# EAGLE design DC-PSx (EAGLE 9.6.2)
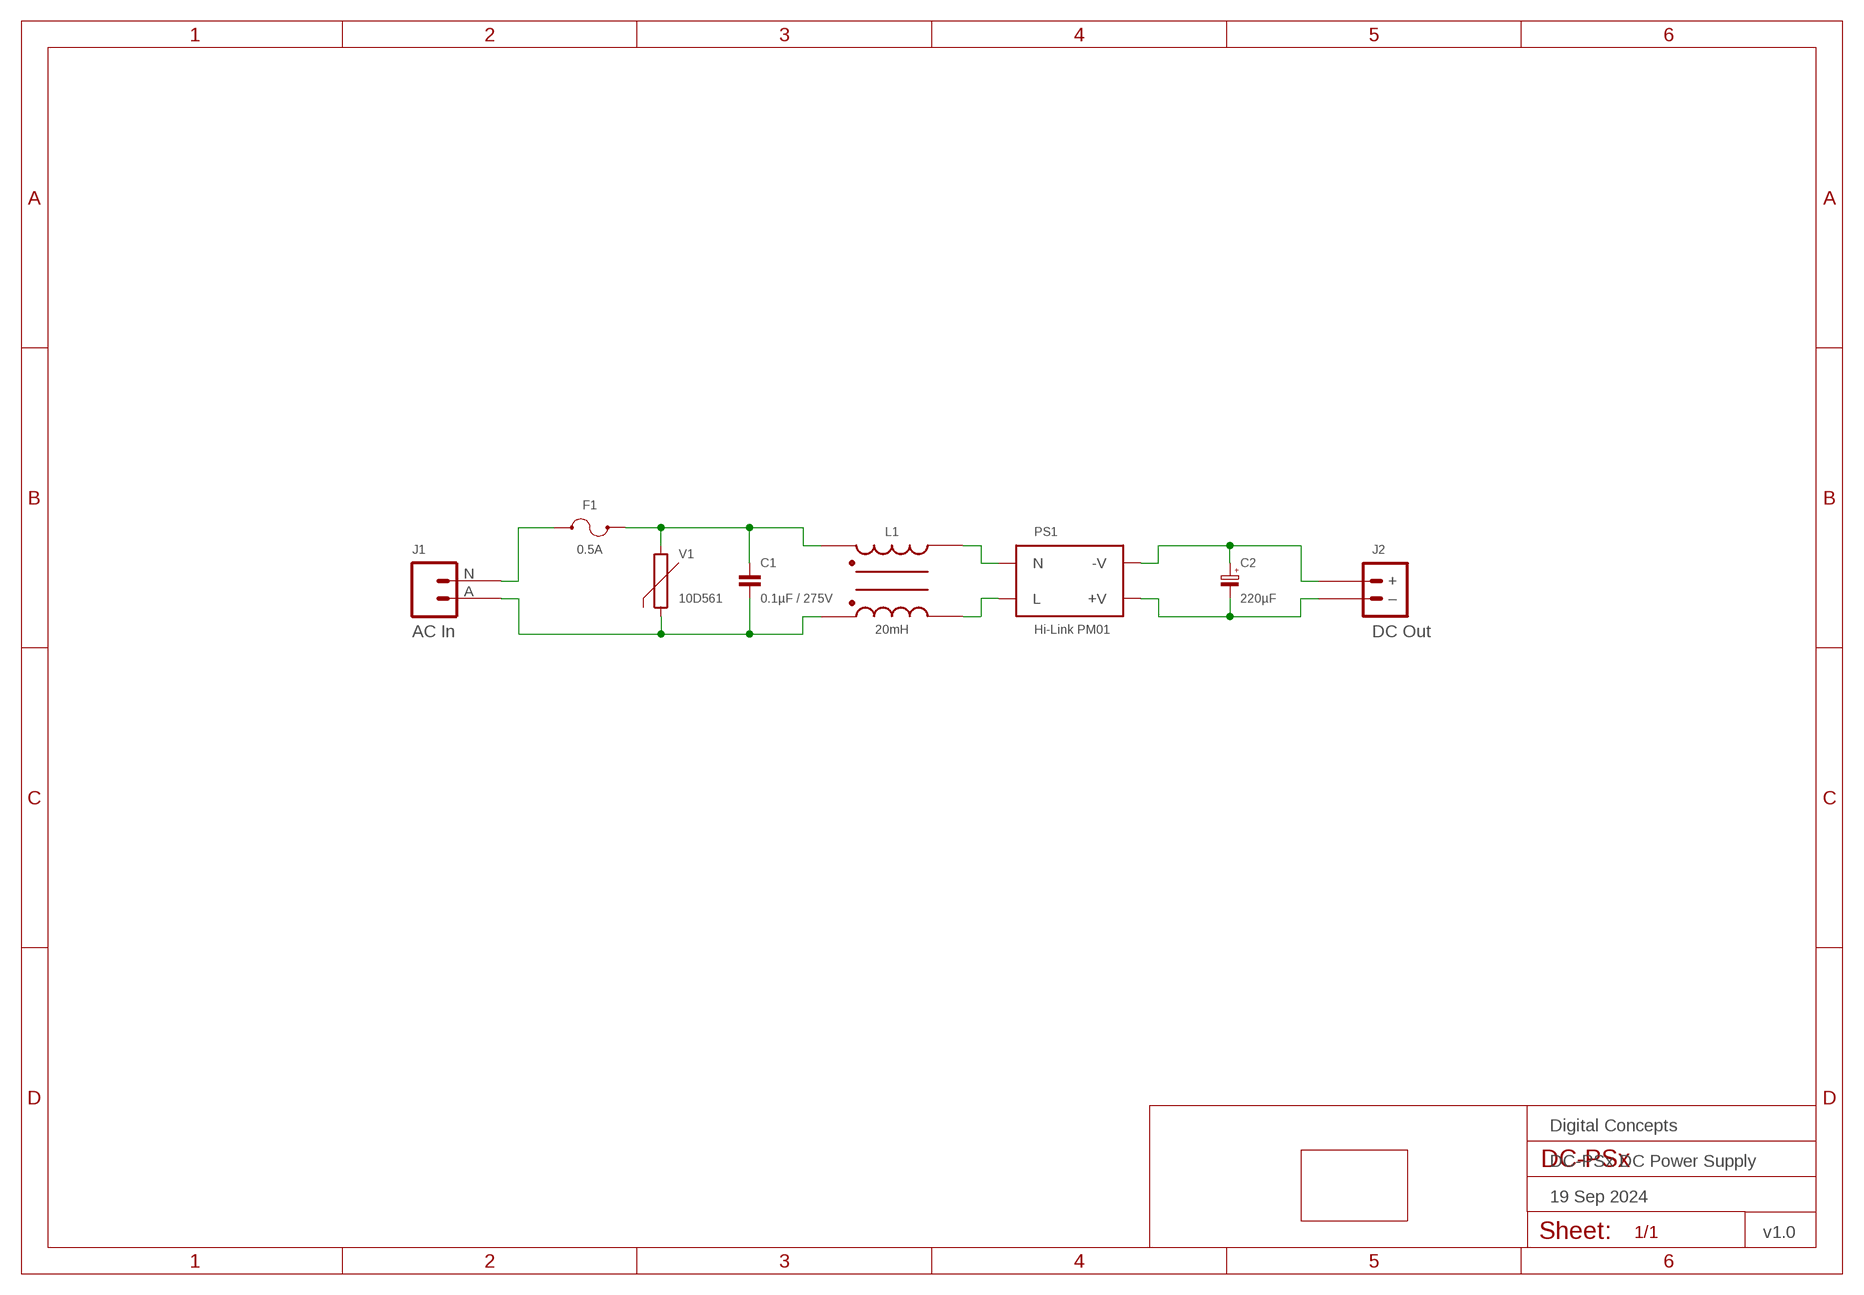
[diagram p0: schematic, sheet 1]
FRAME2 (FRAME-A4L-LOC): DATE: 19 Sep 2024; OWNER: Digital Concepts; TITLE: DC-PSx DC Power Supply; VERSION: v1.0

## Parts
C1  0.1µF / 275V  CAPACITOR-TENTA-SUPPRESSION  [CAPACITOR-TENTA-SUPPRESSION]
C2  220µF  CAPACITOR-ELECTROLYTICE5-10.5  [E5-10,5]
F1  0.5A  FUSE-HOLDER-1808  [FUSE-HOLDER-1808]
J1  AC In  AC_POWER_SOCKET_DB-03  [DB-03_AC_POWER_SOCKET]
J2  DC Out  JST-PH2.0-2-VERTICAL-POWER  [JST-PH2.0-2-VERTICAL-POWER]
L1  20mH  INDUCTOR-COMMON-MODE-UU9.8  [INDUCTOR-UU9.8]
PCB1  PCB-OUTLINE-64X36  [PCB-POWER-SUPPLY-3]
PS1  Hi-Link PM01  POWER_SUPPLY-HI-LINK  [HI-LINK_PM0X]
V1  10D561  VARISTOR-10D561  [VARISTOR-10D561]

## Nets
N$1: F1.P$1 J1.N
N$2: C1.P$1 F1.P$2 L1.P$1 V1.2
N$3: L1.P$2 PS1.AC-N(N)
N$4: C1.P$2 J1.A L1.P$4 V1.1
N$5: L1.P$3 PS1.AC-L(L)
N$6: C2.+ J2.+ PS1.-VO(-V)
N$7: C2.- J2.-(–) PS1.+VO(+V)

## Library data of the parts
C1 = digitalconcepts:CAPACITOR-TENTA-SUPPRESSION: MEX/TENTA Interference Suppression Capacitor
C2 = digitalconcepts:CAPACITOR-ELECTROLYTIC: Electrolytic Capacitor; SPICEPREFIX: C
F1 = digitalconcepts:FUSE-HOLDER-1808: 1808 Fuse Holder
J1 = digitalconcepts:AC_POWER_SOCKET_DB-03: DB-03 AC Power Socket
J2 = digitalconcepts:JST-PH2.0-2-VERTICAL-POWER: JST PH2.0 2P PTH Connector (Power)
L1 = digitalconcepts:INDUCTOR-COMMON-MODE-UU9.8: UU9.8 Common Mode Inductor
PCB1 = digitalconcepts:PCB-OUTLINE-64X36: Power Supply PCB Outline (64 x 36)
PS1 = digitalconcepts:POWER_SUPPLY-HI-LINK: Hi-Link Power Supply Module
V1 = digitalconcepts:VARISTOR-10D561: VARISTOR

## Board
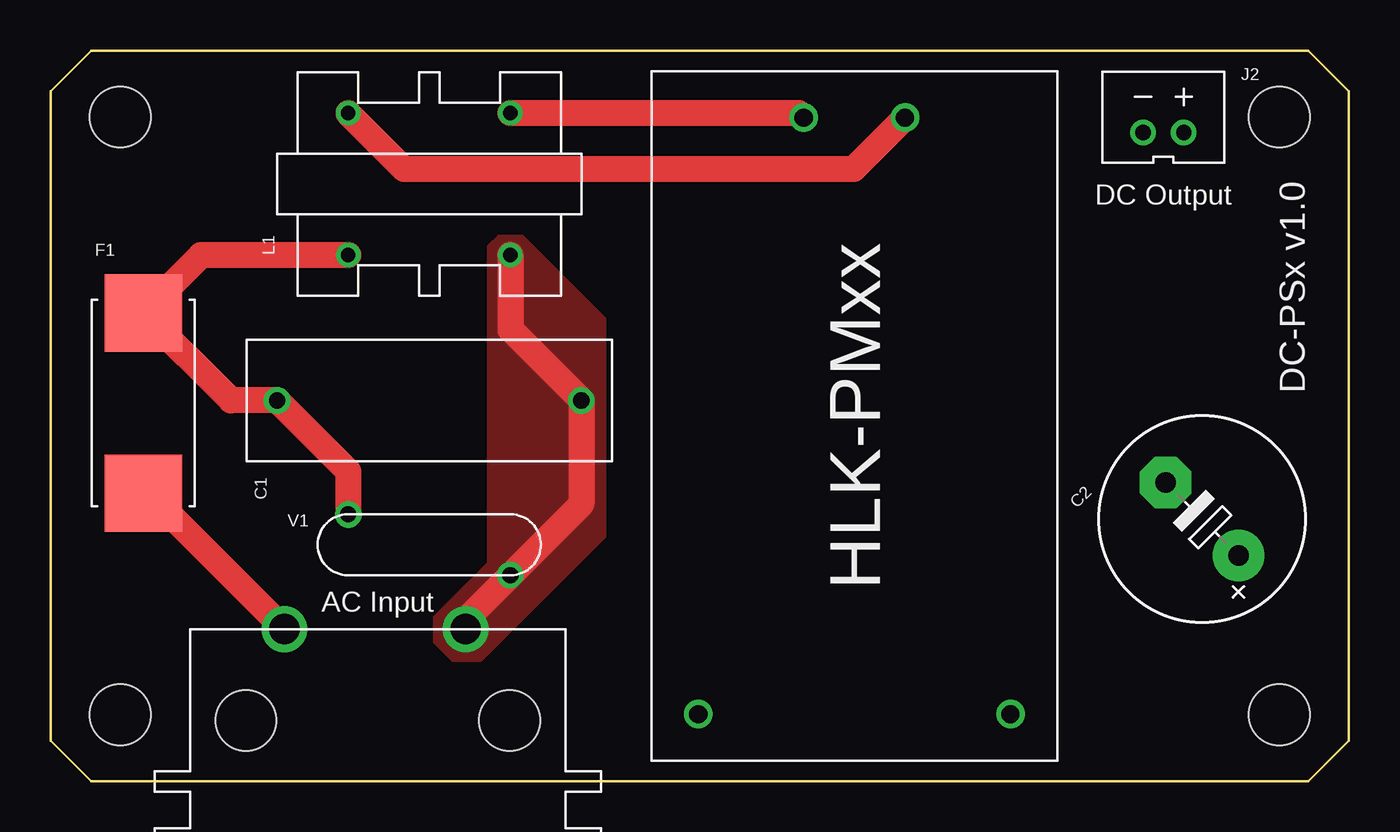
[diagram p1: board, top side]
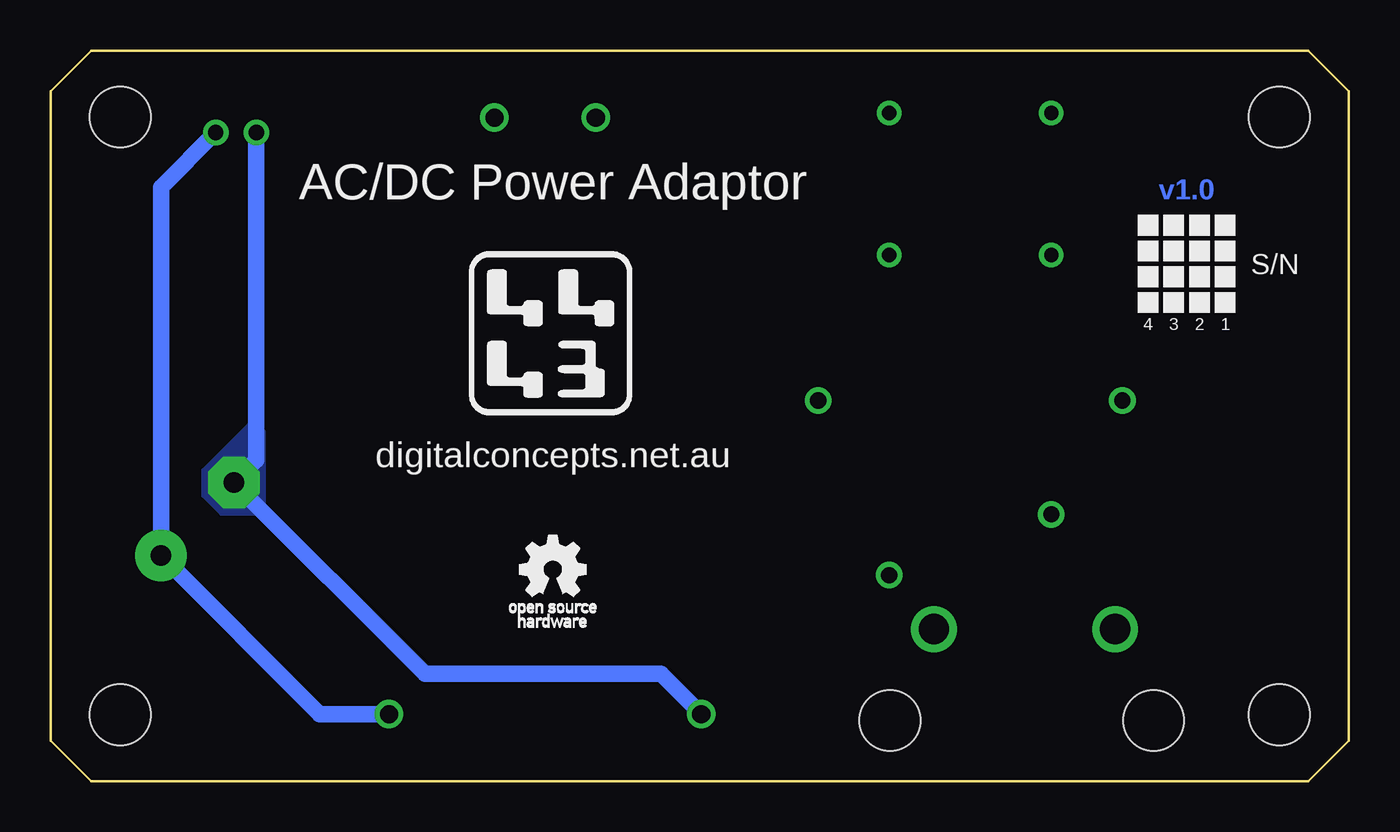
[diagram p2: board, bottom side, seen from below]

Size 64 x 36 mm. Coordinates in mm from the lower left corner, seen from the top.
Copper layers (1*16): Top 0.035mm / dielectric 1.5mm / Bottom 0.035mm
Design rules "default *": minimum track width 6mil, minimum drill 0.35mm, track to track 6mil, track to pad 6mil, pad to pad 6mil, via to via 6mil, smd to smd 6mil, copper to edge 6mil, drill to drill 6mil, minimum pad ring 10mil, minimum via ring 8mil, stop-mask expansion 4mil, vias tented up to drill 0mil, thermal gap 10mil

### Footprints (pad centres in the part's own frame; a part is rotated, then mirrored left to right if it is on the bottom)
CAPACITOR-TENTA-SUPPRESSION = drill 0.8: P$1 -7.5,0; P$2 7.5,0
E5-10,5 = drill 1.016 pad 2.54: + -2.54,0 | drill 1.016 pad 2.54 octagon: - 2.54,0
FUSE-HOLDER-1808 = smd 3.81 x 3.81: P$1 -4.445,0; P$2 4.445,0
DB-03_AC_POWER_SOCKET = drill 1.5: A -4.33,-6; N 4.6,-6 | hole 3: -6.5,-1.5; 6.5,-1.5
JST-PH2.0-2-VERTICAL-POWER = drill 0.75: + -1,0; - 1,0
INDUCTOR-UU9.8 = drill 0.7: P$1 -3.5,4; P$2 3.5,4; P$3 3.5,-4; P$4 -3.5,-4
PCB-POWER-SUPPLY-3 = hole 3: -28.575,14.732; -28.575,-14.732; 28.575,-14.732; 28.575,14.732
HI-LINK_PM0X = drill 0.9: +VO 14.7,-7.7; -VO 14.7,7.7; AC-L -14.7,-2.5; AC-N -14.7,2.5
VARISTOR-10D561 = drill 0.8: 1 -4,1.5; 2 4,-1.5

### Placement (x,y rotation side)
C1  18.66,18.76 0 top
C2  56.77,12.92 135 top
F1  4.57,18.64 90 top
J1  16.12,1.49 180 top
J2  54.86,31.97 180 top
L1  18.66,29.43 90 top
PCB1  32,18 0 top
PS1  39.62,18 270 top
V1  18.66,11.65 180 top

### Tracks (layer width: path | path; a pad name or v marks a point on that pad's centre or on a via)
N$1
  Top 1.27: F1.P$1 4.82,14.19 J1.N
N$2
  Top 1.27: V1.2 14.66,15.26 C1.P$1 8.89,18.76 F1.P$2 7.42,25.93 L1.P$1
N$3
  Top 1.27: PS1.AC-N 39.58,30.16 17.43,30.16 L1.P$2
N$4
  Top 1.27: L1.P$4 22.66,22.26 C1.P$2 26.16,13.65 V1.1 20.45,7.94 J1.A
  pour Top (no thermals): 22.09,26.89 23.24,26.89 27.3,22.83 27.3,12.03 21.2,5.94 19.81,5.94 18.92,6.82 18.92,8.09 21.59,10.76 21.59,26.38
N$5
  Top 1.27: PS1.AC-L 36.89,32.93 L1.P$3
N$6
  Bottom 0.813: PS1.-VO 50.74,3.3 C2.+ 58.56,29.27 J2.+
N$7
  Bottom 0.813: PS1.+VO 33.92,5.3 45.55,5.3 C2.- 53.86,15.83 J2.-
  pour Bottom (no thermals): 53.46,17.24 53.84,17.62 54.23,17.62 56.51,15.33 56.51,14.06 55.62,13.17 53.84,13.17 53.46,13.55

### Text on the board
Bottom: v1.0
tPlace: DC-PSx v1.0
bPlace: AC/DC Power Adaptor | S/N | 1 | 2 | 3 | 4 | digitalconcepts.net.au
tNames: DC Output | AC Input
